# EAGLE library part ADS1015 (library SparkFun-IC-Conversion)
ADS1015 12-BIT ADC 12-Bit Del-Sig ADC Four single-ended inputs or two differential inputs Internal PGA I2C interface 2.0-5.5V SparkFun Products SparkFun Block for Intel Edison - ADC (DEV-13770)
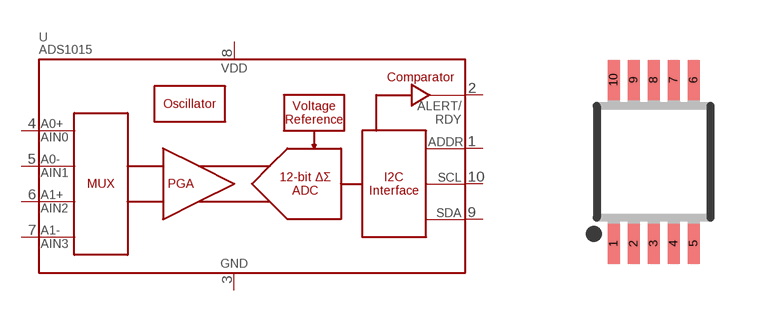
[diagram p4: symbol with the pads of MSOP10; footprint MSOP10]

Designator prefix U

## ADS1015 (PROD_ID: IC-12270; VALUE: ADS1015)  [MSOP10]
1  ADDR
2  ALERT/RDY
3  VSS
4  AIN0
5  AIN1
6  AIN2
7  AIN3
8  VDD
9  SDA
10  SCL

## Footprint MSOP10 (pad centres in mm)
10 Lead Platic MSOP Source: http://www.linear.com .. LT1996
smd 0.3 x 1: 1 -1,-2.05; 2 -0.5,-2.05; 3 0,-2.05; 4 0.5,-2.05; 5 1,-2.05; 6 1,2.05; 7 0.5,2.05; 8 0,2.05; 9 -0.5,2.05; 10 -1,2.05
